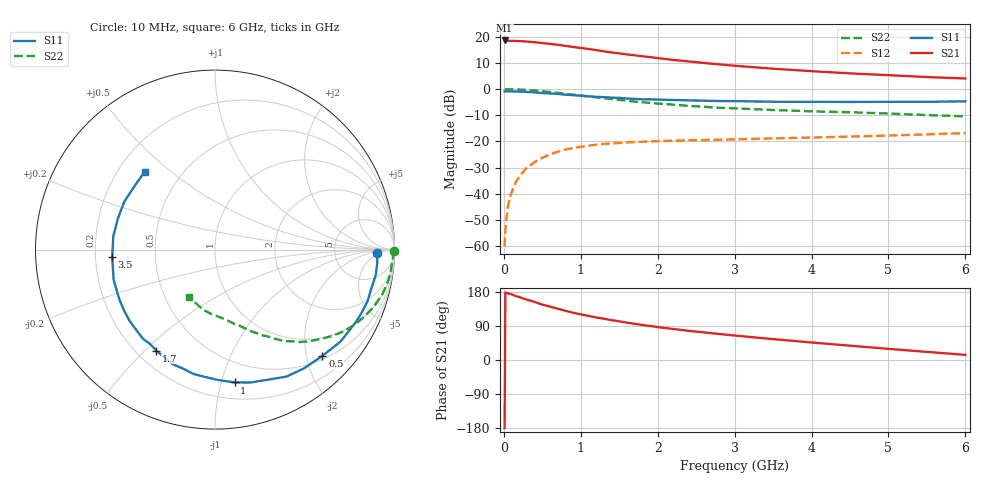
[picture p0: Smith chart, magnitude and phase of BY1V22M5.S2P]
! SIEMENS Small Signal Semiconductors
! BFY420
! Si NPN RF SIEGET Grounded Emitter Transistor in MICRO-X
! VCE = 1.25 V  IC = 2.5 mA
! Common Emitter S-Parameters:  October  1996
# GHz  S  MA  R  50
!  f  S11  S21  S12  S22
! GHz  MAG  ANG  MAG  ANG  MAG  ANG  MAG  ANG
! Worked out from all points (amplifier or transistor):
!   36 points, 10 MHz to 6 GHz, reference 50 ohm
!   highest |S21| = 18.6 dB at 10 MHz (marker M1)
!   |S21| within 3 dB of that: start of sweep to 1.033 GHz
!   unconditionally stable (mu >= 1): 3.781 GHz to end of sweep
!   at 250 MHz: K = 0.06, MSG = 25.0 dB, |S12| = -31.6 dB
!   at 1.4 GHz: K = 0.35, MSG = 17.4 dB, |S12| = -20.8 dB
!   at 6 GHz: K = 1.24, MAG = 7.5 dB, |S12| = -16.8 dB
!   S11 on the Smith chart (normalised r, x): 10 MHz: 19, -4; 500 MHz: 0.57, -2.31; 1 GHz: 0.33, -1.10; 1.7 GHz: 0.28, -0.54; 3.5 GHz: 0.27, -0.03; 6 GHz: 0.31, +0.41
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0.01  0.9032 -1.2  8.499 -179.7  0.001 99.8  0.9947 -0.5
0.02  0.9037 -1.8  8.465 178.3  0.0021 84.8  0.9883 -0.9
0.05  0.9074 -4.7  8.35 176.0  0.0055 88.4  0.9931 -2.5
0.1  0.9065 -9.2  8.35 173.5  0.0106 86.2  0.9879 -5.1
0.15  0.8979 -13.8  8.287 168.9  0.0161 81.1  0.9866 -7.6
0.2  0.8973 -18.5  8.26 166.3  0.0212 80.4  0.9812 -10.0
0.25  0.8901 -23.1  8.2 162.5  0.0262 76.4  0.9723 -12.7
0.4  0.8672 -36.2  7.88 153.3  0.0403 69.5  0.9398 -19.8
0.5  0.8417 -44.7  7.57 146.1  0.0487 64.9  0.9112 -24.3
0.7  0.8115 -60.7  7.024 135.3  0.0636 56.2  0.85 -32.3
0.9  0.7667 -74.9  6.382 124.8  0.075 48.8  0.7831 -39.0
1  0.7481 -81.6  6.1 120.5  0.0791 45.9  0.7521 -42.1
1.1  0.7271 -88.5  5.852 116.4  0.0832 42.9  0.724 -45.0
1.4  0.6865 -105.0  5.005 105.2  0.0917 35.9  0.6473 -52.0
1.7  0.651 -120.1  4.431 95.5  0.0974 30.6  0.5771 -57.7
2  0.6304 -132.6  3.918 86.9  0.1016 26.8  0.5289 -62.4
2.2  0.6202 -139.9  3.619 81.9  0.1033 24.4  0.5055 -65.3
2.8  0.5922 -158.2  2.971 68.6  0.108 20.1  0.4402 -72.9
3.5  0.5742 -176.1  2.454 55.1  0.1145 17.1  0.3988 -80.4
4.5  0.5682 162.0  1.997 37.8  0.1237 13.8  0.3611 -92.7
5.5  0.5714 141.3  1.699 21.4  0.1368 11.0  0.3193 -108.7
6  0.5846 132.2  1.595 13.5  0.1444 9.3  0.302 -118.3
